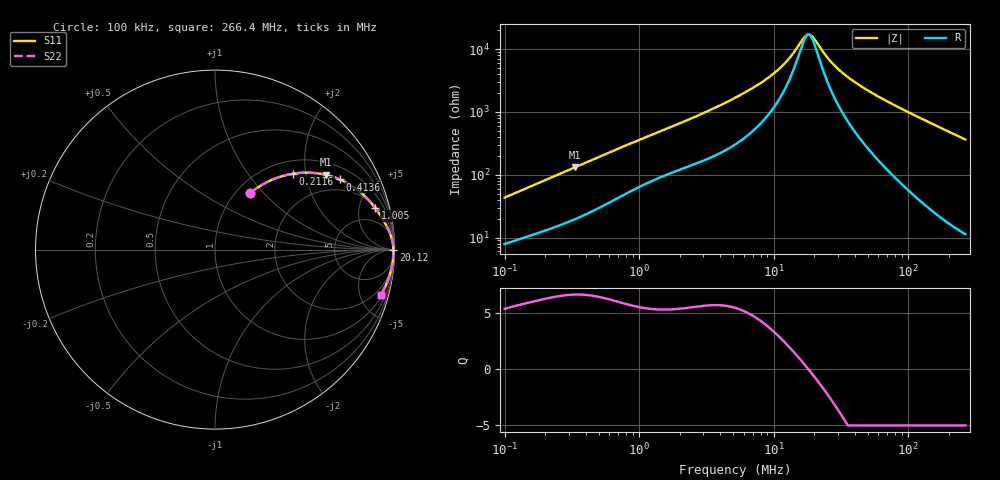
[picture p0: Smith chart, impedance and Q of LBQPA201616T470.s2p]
! LBQPA201616T470  S-PARAMETER MODEL  ( General Type )
! Model Generated by TAIYO YUDEN Corporation (http://www.ty-top.com)
! Version 1.0
! TAIYO YUDEN Control No. 191025NI43SB-FBB
! Copyright(c) 2019 TAIYO YUDEN CO.,LTD. All Rights Reserved.
! Product Description (link to TY-COMPAS)
! https://ds.yuden.co.jp/TYCOMPAS/or/detail?pn=LBQPA201616T470K&u=M
! Products Name : Inductors
! Characteristics :
!  Inductance : 47 uH , SRF(min) : 11 MHz , DC Resistance(max) : 5.59 Ohm
!  Rated Current : Saturation :150 mA , Temp Rise : 130 mA (20 degC)
!  Case Size : 2.0 x 1.6 / 0.079 x 0.063 [mm/inch] , Thickness : 1.6 / 0.063 [mm/inch]
!  (Conditions: Temperature = 25 degC , DC Bias Current/Voltage = 0A / 0V)
! External Node Assignments :
!  1  o---GGG---o  2
! GND o---------o GND
! Frequency Range : 0.1MHz  -  266.375554MHz  [ 402 STEP ]
# MHz S RI R 50
! Freq[MHz].  S11 Real  S11 Imag  S21 Real  S21 Imag  S12 Real  S12 Imag  S22 Real  S22 Imag
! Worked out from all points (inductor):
!   401 points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, 100 kHz to 266.4 MHz, reference 50 ohm
!   read as one part in series: L = 66.4 uH near 104 kHz
!   highest Q = 6.64 at 333 kHz (marker M1), where L = 62 uH
!   self-resonance near 17.88 MHz
!   S11 on the Smith chart (normalised r, x): 100 kHz: 1.16, +0.85; 211.6 kHz: 1.27, +1.70; 413.6 kHz: 1.48, +3.18; 1.005 MHz: 2.28, +7.08; 20.12 MHz: open; 266.4 MHz: 1.23, -7.27
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0.1  0.1976 0.3159  0.8024 -0.3159  0.8024 -0.3159  0.1976 0.3159
0.211554  0.4357 0.4231  0.5643 -0.4231  0.5643 -0.4231  0.4357 0.4231
0.332957  0.6161 0.4169  0.3839 -0.4169  0.3839 -0.4169  0.6161 0.4169
0.374775  0.6602 0.4043  0.3398 -0.4043  0.3398 -0.4043  0.6602 0.4043
0.413608  0.6947 0.3909  0.3053 -0.3909  0.3053 -0.3909  0.6947 0.3909
0.625788  0.8114 0.3183  0.1886 -0.3183  0.1886 -0.3183  0.8114 0.3183
1.004517  0.8922 0.2326  0.1078 -0.2326  0.1078 -0.2326  0.8922 0.2326
1.404561  0.9272 0.1822  0.0728 -0.1822  0.0728 -0.1822  0.9272 0.1822
2.913391  0.9711 0.1007  0.0289 -0.1007  0.0289 -0.1007  0.9711 0.1007
5.26394  0.9864 0.0559  0.0136 -0.0559  0.0136 -0.0559  0.9864 0.0559
9.893512  0.9925 0.0235  0.00752 -0.0235  0.00752 -0.0235  0.9925 0.0235
12.78436  0.9935 0.0131  0.00649 -0.0131  0.00649 -0.0131  0.9935 0.0131
17.18443  0.9941 0.002  0.00586 -0.002  0.00586 -0.002  0.9941 0.002
18.23166  0.9942 -0.000186  0.00579 0.000186  0.00579 0.000186  0.9942 -0.000186
19.34272  0.9943 -0.00238  0.00573 0.00238  0.00573 0.00238  0.9943 -0.00238
20.12079  0.9943 -0.00384  0.00571 0.00384  0.00571 0.00384  0.9943 -0.00384
25.49235  0.9943 -0.0129  0.0057 0.0129  0.0057 0.0129  0.9943 -0.0129
32.29792  0.994 -0.0226  0.00595 0.0226  0.00595 0.0226  0.994 -0.0226
45.16044  0.9931 -0.0387  0.0069 0.0387  0.0069 0.0387  0.9931 -0.0387
72.49162  0.9897 -0.0693  0.0103 0.0693  0.0103 0.0693  0.9897 -0.0693
141.7277  0.9738 -0.1398  0.0262 0.1398  0.0262 0.1398  0.9738 -0.1398
266.3756  0.9231 -0.2514  0.0769 0.2514  0.0769 0.2514  0.9231 -0.2514
